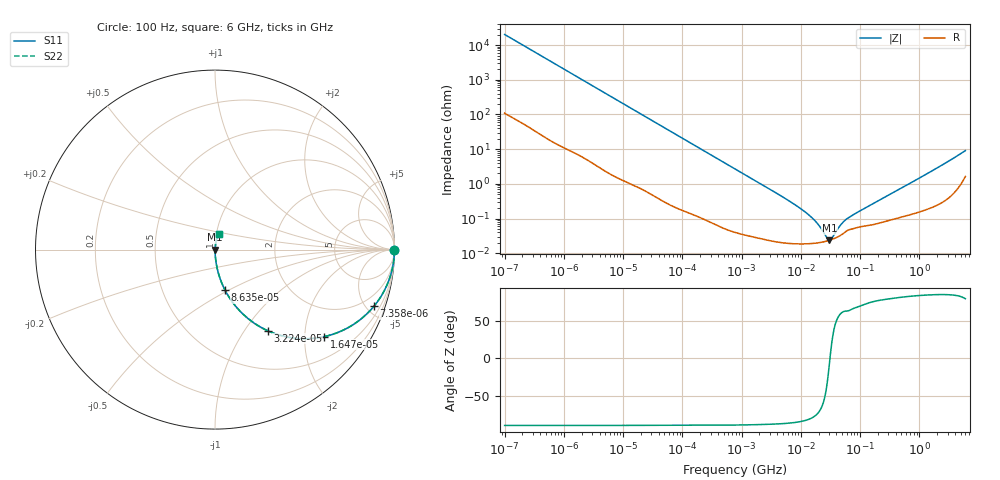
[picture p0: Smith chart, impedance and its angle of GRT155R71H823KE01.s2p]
!Murata Part Number: GRT155R71H823KE01
!These Parameters are Measured in Series Mode Connection
!Data Generated on Jun 19, 2026
!  o--ll--o
!Port1  Port2
!  o------o
!Operation Temp=25[degC], DC Bias Voltage=0[V]
!Freq. Start=100[Hz] Stop=6[GHz] 401[Steps]
# Hz S RI R 50
!Freq.(Hz) S11(Real) S11(Imag) S21(Real) S21(Imag) S12(Real) S12(Imag) S22(Real) S22(Imag)
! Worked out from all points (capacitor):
!   401 points, 100 Hz to 6 GHz, reference 50 ohm
!   read as one part in series: C = 78.4 nF near 109 Hz
!   lowest |Z| = 23.7 mohm at 30.45 MHz (marker M1)
!   series resonance near 31.07 MHz, so ESL is about 330 pH
!   S11 on the Smith chart (normalised r, x): 100 Hz: open; 7.358 kHz: 1.03, -5.59; 16.47 kHz: 1.02, -2.50; 32.24 kHz: 1.01, -1.28; 86.35 kHz: 1.00, -0.48; 6 GHz: 1.03, +0.18
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100  0.9999 -0.00494  5.1e-05 0.00494  5.1e-05 0.00494  0.9999 -0.00494
627  0.9989 -0.0307  0.0011 0.0307  0.0011 0.0307  0.9989 -0.0307
2008  0.9899 -0.0971  0.0101 0.0971  0.0101 0.0971  0.9899 -0.0971
4299  0.9569 -0.2002  0.0431 0.2002  0.0431 0.2002  0.9569 -0.2002
7358  0.8851 -0.3161  0.1149 0.3161  0.1149 0.3161  0.8851 -0.3161
11009  0.7762 -0.4137  0.2238 0.4137  0.2238 0.4137  0.7762 -0.4137
16473  0.6097 -0.4844  0.3903 0.4844  0.3903 0.4844  0.6097 -0.4844
32244  0.293 -0.4516  0.707 0.4516  0.707 0.4516  0.293 -0.4516
40335  0.2103 -0.404  0.7897 0.404  0.7897 0.404  0.2103 -0.404
86348  0.0563 -0.2265  0.9437 0.2265  0.9437 0.2265  0.0563 -0.2265
221108  0.00979 -0.0934  0.9902 0.0934  0.9902 0.0934  0.00979 -0.0934
774597  0.00113 -0.0271  0.9989 0.0271  0.9989 0.0271  0.00113 -0.0271
6644369  0.000199 -0.00305  0.9998 0.00305  0.9998 0.00305  0.000199 -0.00305
1.555665e7  0.000192 -0.00102  0.9998 0.00102  0.9998 0.00102  0.000192 -0.00102
2.035112e7  0.000201 -0.000594  0.9998 0.000594  0.9998 0.000594  0.000201 -0.000594
2.784235e7  0.000225 -0.000149  0.9998 0.000149  0.9998 0.000149  0.000225 -0.000149
3.045065e7  0.000236 -2.68e-05  0.9998 2.68e-05  0.9998 2.68e-05  0.000236 -2.68e-05
3.330331e7  0.000248 9.4e-05  0.9998 -9.4e-05  0.9998 -9.4e-05  0.000248 9.4e-05
4.556224e7  0.000318 0.000519  0.9997 -0.000519  0.9997 -0.000519  0.000318 0.000519
5.960426e7  0.000442 0.000873  0.9996 -0.000873  0.9996 -0.000873  0.000442 0.000873
3.124326e8  0.000911 0.00481  0.9991 -0.00481  0.9991 -0.00481  0.000911 0.00481
6e9  0.0236 0.0858  0.9764 -0.0858  0.9764 -0.0858  0.0236 0.0858
